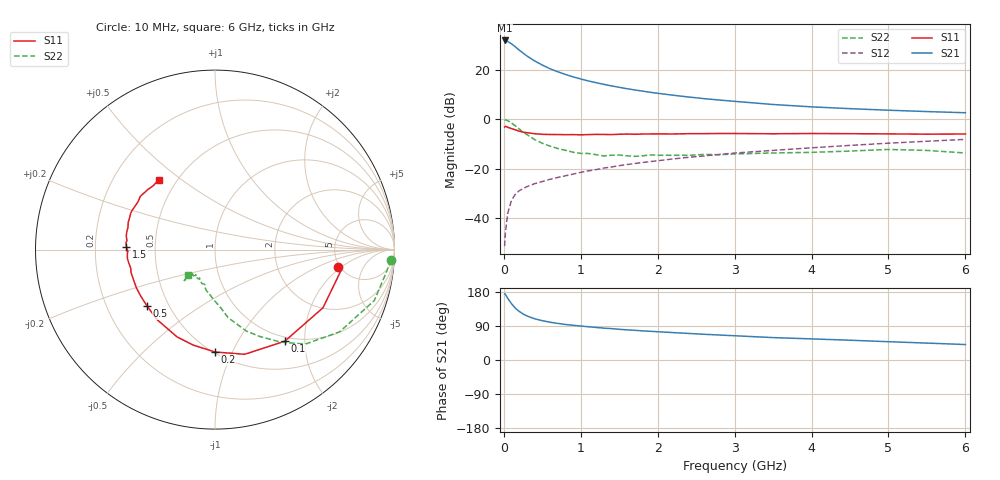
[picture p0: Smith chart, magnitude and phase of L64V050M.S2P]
!  INFINEON TECHNOLOGIES Small Signal Semiconductors
! BFR380L3 , Si-NPN RF-Transistor in TSLP-3-1
!  Vce=4 V,  Ic=50 mA
! Common Emitter S-Parameters:  07. March 2005
#  GHz  S  MA  R  50
! f  S11  S21  S12  S22
! GHz  Mag  Ang  Mag  Ang  Mag  Ang  Mag  Ang
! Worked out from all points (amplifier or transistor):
!   36 points, 10 MHz to 6 GHz, reference 50 ohm
!   highest |S21| = 31.8 dB at 10 MHz (marker M1)
!   |S21| within 3 dB of that: start of sweep to 165.9 MHz
!   unconditionally stable (mu >= 1): 1.688 GHz to 4.819 GHz
!   at 250 MHz: K = 0.43, MSG = 27.4 dB, |S12| = -28.1 dB
!   at 1.4 GHz: K = 0.98, MSG = 16.4 dB, |S12| = -19.4 dB
!   at 6 GHz: K = 0.97, MSG = 5.4 dB, |S12| = -8.2 dB
!   S11 on the Smith chart (normalised r, x): 10 MHz: 4.75, -1.78; 100 MHz: 0.93, -1.61; 200 MHz: 0.51, -0.86; 500 MHz: 0.38, -0.32; 1.5 GHz: 0.34, +0.01; 6 GHz: 0.40, +0.41
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0.01  0.6899 -8.2  38.81 174.6  0.0027 84.0  0.9798 -3.3
0.02  0.7141 -8.8  38.52 173.3  0.005 87.4  0.9649 -7.1
0.05  0.6834 -28.3  37.12 162.9  0.0124 80.3  0.932 -17.7
0.1  0.6417 -52.7  33.12 148.4  0.0228 67.5  0.832 -33.4
0.15  0.6062 -74.2  28.82 136.7  0.0305 61.2  0.7283 -46.3
0.2  0.5705 -90.0  24.8 128.1  0.0356 58.5  0.6312 -54.7
0.25  0.5456 -102.9  21.58 121.6  0.0395 55.0  0.543 -62.9
0.3  0.5304 -113.5  18.85 116.3  0.0431 54.9  0.4855 -69.0
0.4  0.5064 -129.5  14.99 108.8  0.0495 53.8  0.3858 -79.1
0.5  0.4923 -140.2  12.35 103.8  0.0547 55.0  0.3237 -84.6
0.6  0.488 -148.3  10.42 99.7  0.0606 56.0  0.2847 -90.5
0.7  0.487 -154.0  9.054 96.6  0.0661 57.8  0.2544 -96.2
0.8  0.4841 -159.9  7.987 93.8  0.0714 59.2  0.234 -101.7
0.9  0.4851 -164.8  7.124 91.6  0.0771 60.0  0.2137 -105.7
1.1  0.486 -171.1  5.9 87.6  0.0899 62.2  0.2019 -111.4
1.5  0.4934 178.3  4.385 81.0  0.1145 64.3  0.1875 -121.5
1.8  0.4984 172.1  3.676 76.9  0.1325 64.9  0.18 -126.8
2.2  0.5002 165.8  3.035 72.3  0.1564 65.1  0.1851 -129.9
3.5  0.5049 148.1  1.971 59.1  0.2329 63.4  0.2068 -135.7
4.5  0.5067 142.0  1.624 52.2  0.2938 61.8  0.2258 -135.2
5.5  0.4949 133.9  1.418 44.6  0.3563 58.2  0.2325 -134.9
6  0.4995 128.9  1.343 40.8  0.3889 56.1  0.2064 -136.5
